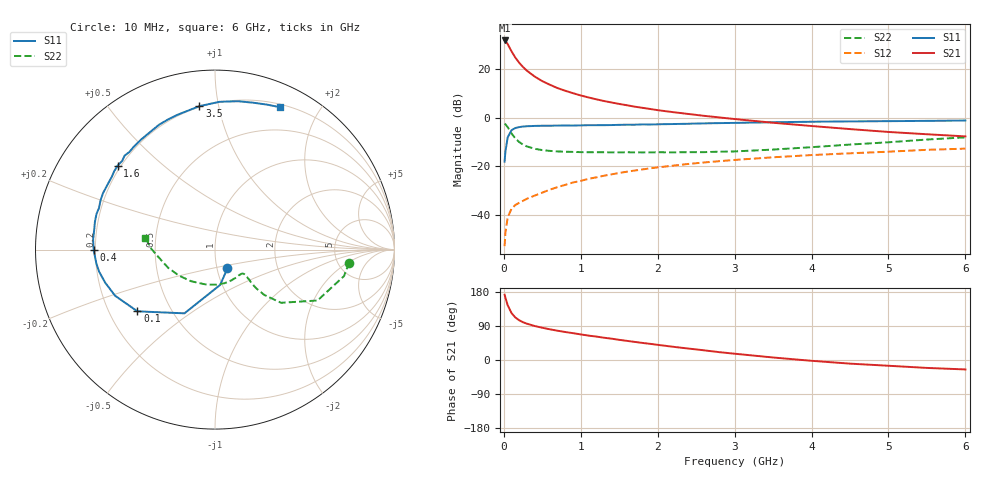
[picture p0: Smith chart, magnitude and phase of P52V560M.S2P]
! SIEMENS Small Signal Semiconductors
! BFP183
! Si NPN RF Bipolar Junction Transistor in SOT143
! VCE = 2.5 V  IC = 60 mA
! Common Emitter S-Parameters:  March  1996
# GHz  S  MA  R  50
!  f  S11  S21  S12  S22
! GHz  MAG  ANG  MAG  ANG  MAG  ANG  MAG  ANG
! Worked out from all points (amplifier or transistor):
!   36 points, 10 MHz to 6 GHz, reference 50 ohm
!   highest |S21| = 31.7 dB at 10 MHz (marker M1)
!   |S21| within 3 dB of that: start of sweep to 75.16 MHz
!   unconditionally stable (mu >= 1): start of sweep to 32.64 MHz; 187.8 MHz to end of sweep
!   at 250 MHz: K = 1.15, MAG = 25.1 dB, |S12| = -34.2 dB
!   at 1.4 GHz: K = 1.68, MAG = 9.9 dB, |S12| = -23.3 dB
!   at 6 GHz: K = 1.26, MAG = -0.5 dB, |S12| = -12.7 dB
!   S11 on the Smith chart (normalised r, x): 10 MHz: 1.12, -0.24; 100 MHz: 0.32, -0.32; 400 MHz: 0.19, -0.00; 1.6 GHz: 0.19, +0.36; 3.5 GHz: 0.19, +0.88; 6 GHz: 0.23, +1.53
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0.01  0.1253 -56.5  38.37 172.2  0.0023 63.3  0.7511 -5.5
0.02  0.1986 -81.6  37.52 164.6  0.0043 69.8  0.7338 -11.6
0.05  0.3938 -115.6  32.29 144.4  0.009 62.9  0.6377 -26.4
0.1  0.5524 -141.5  22.9 123.8  0.0135 47.3  0.473 -38.8
0.15  0.6131 -155.2  17.02 112.1  0.0161 45.7  0.3732 -42.6
0.2  0.6388 -163.2  13.35 104.8  0.0179 48.1  0.315 -43.2
0.25  0.6571 -169.2  10.9 99.6  0.0196 49.5  0.2797 -42.6
0.3  0.6651 -173.1  9.193 95.8  0.0216 52.3  0.2563 -41.5
0.4  0.676 -179.7  6.993 89.7  0.0251 55.1  0.2295 -40.3
0.5  0.6814 175.1  5.605 85.1  0.0289 57.3  0.2156 -40.0
0.6  0.6818 170.9  4.721 80.9  0.0333 59.2  0.2077 -40.3
0.7  0.6866 167.0  4.026 77.2  0.0376 60.5  0.2023 -41.2
0.9  0.6866 160.3  3.172 70.8  0.0467 61.5  0.1978 -44.5
1.1  0.6987 153.3  2.597 64.4  0.0554 61.7  0.195 -48.6
1.3  0.7004 147.9  2.194 58.8  0.0641 61.0  0.1947 -53.6
1.6  0.7165 139.2  1.796 50.5  0.0777 59.0  0.1945 -61.4
2.2  0.7388 123.8  1.296 34.9  0.1034 53.7  0.1938 -80.5
2.8  0.7715 109.6  1.01 20.7  0.1276 47.4  0.1999 -101.8
3.5  0.804 96.2  0.785 6.6  0.1535 40.3  0.2211 -127.3
4.5  0.8367 81.1  0.582 -9.6  0.1853 30.0  0.28 -158.8
5.5  0.8581 70.3  0.456 -20.9  0.2183 20.6  0.355 179.3
6  0.8715 65.6  0.412 -24.9  0.231 15.4  0.3939 170.4
